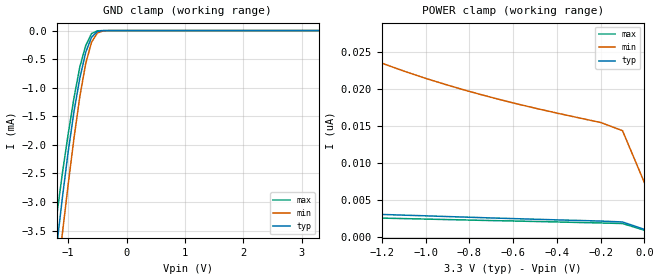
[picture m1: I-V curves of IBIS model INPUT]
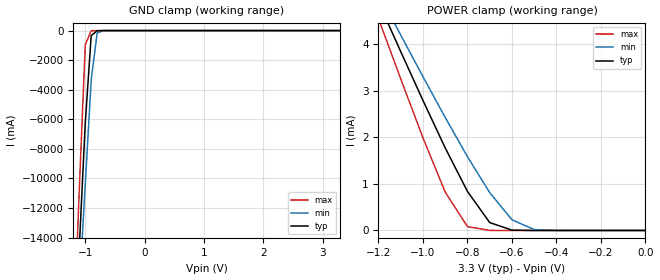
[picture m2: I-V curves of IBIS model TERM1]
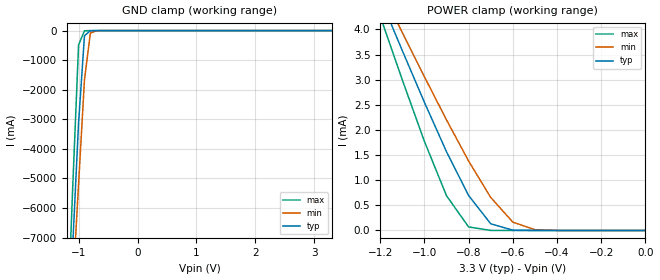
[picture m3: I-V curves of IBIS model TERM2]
|   DIODES INCORPORATED
|   IBIS Model of PI3B33X257
|   Product Family: 3B
|   BQSOP (B) Package
[IBIS Ver] 3.2
[Comment char] |_char
[File Name] pi3b33x257_b_33v.ibs
[File Rev] 1.0
[Source] File originated at Diodes Incorporated.
[Date] 10/15/15
[Disclaimer] (C) Copyright DIODES INCORPORATED
   All rights reserved
  Diodes Incorporated hereby grants the user of
  this IBIS model a non-exclusive, nontransferable license to
  use this IBIS model under the following terms.
  This IBIS model is provided on an "AS IS" basis and Diodes
  makes absolutely no warranty with respect to the information
  contained herein. DIODES DISCLAIMS AND CUSTOMER WAIVES ALL
  WARRANTIES, EXPRESSED OR IMPLIED, INCLUDING WARRANTIES OF
  MERCHANTABILITY OR FITNESS FOR A PARTICULAR PURPOSE. The
  entire risk as to quality and performance is with the customer.
  Accordingly, in no event shall the company be liable for any
  damages, whether in contract or tort, including any lost
  profits or other incidental, consequential, exemplary, or
  punitive damages arising out of the use or application of the
  IBIS model provided in this package. Further, Diodes reserves
  the right to make changes without notice to any product herein
  to improve reliability, function, or design. Diodes does not
  convey any license under patent rights or any other intellectual
  property rights, including those of third parties.
  The user is granted this license only to use the IBIS model
  and is not granted rights to sell, load, rent, lease or license
  the IBIS model in whole or in part, or in modified form to anyone
  other than user. User may modify the IBIS model to suit its specific
  application but rights to derivative works and such modifications
  shall belong to Diodes.
  Diodes is not obligated to provide maintenance or support
  for the licensed IBIS model.
  Contact Diodes at ATTN: APPLICATION ENGINEERING / IBIS MODELS
  1545 Barber Ln. Milpitas, CA 95035
[Component] PI3B33X257
[Manufacturer] Diodes Incorporated.
[Package]
| variable   typ   min   max
R_pkg   0.05665ohm   0.05080ohm   0.06250ohm
L_pkg   2.96700nH   2.48200nH   3.45200nH
C_pkg   0.32100pF   0.26800pF   0.37400pF
[Pin]   signal_name   model_name   R_pin   L_pin   C_pin
1   S0   INPUT   0.06250   3.45200nH   0.37400pF
2   IA0   TERM1   0.06144   3.36382nH   0.36436pF
3   IA1   TERM1   0.06037   3.27564nH   0.35473pF
4   YA   TERM2   0.05931   3.18745nH   0.34509pF
5   IB0   TERM1   0.05825   3.09927nH   0.33545pF
6   IB1   TERM1   0.05718   3.01109nH   0.32582pF
7   YB   TERM2   0.05612   2.92291nH   0.31618pF
8   GND   GND   0.05505   2.83473nH   0.30655pF
9   S1   INPUT   0.05399   2.74655nH   0.29691pF
10   IE0   TERM1   0.05293   2.65836nH   0.28727pF
11   IE1   TERM1   0.05186   2.57018nH   0.27764pF
12   YE   TERM2   0.05080   2.48200nH   0.26800pF
13   IF0   TERM1   0.05080   2.48200nH   0.26800pF
14   IF1   TERM1   0.05186   2.57018nH   0.27764pF
15   YF   TERM2   0.05293   2.65836nH   0.28727pF
16   GND   GND   0.05399   2.74655nH   0.29691pF
17   S2   INPUT   0.05505   2.83473nH   0.30655pF
18   II0   TERM1   0.05612   2.92291nH   0.31618pF
19   II1   TERM1   0.05718   3.01109nH   0.32582pF
20   YI   TERM2   0.05825   3.09927nH   0.33545pF
21   IJ0   TERM1   0.05931   3.18745nH   0.34509pF
22   IJ1   TERM1   0.06037   3.27564nH   0.35473pF
23   YJ   TERM2   0.06144   3.36382nH   0.36436pF
24   GND   GND   0.06250   3.45200nH   0.37400pF
25   YK   TERM2   0.06250   3.45200nH   0.37400pF
26   IK1   TERM1   0.06144   3.36382nH   0.36436pF
27   IK0   TERM1   0.06037   3.27564nH   0.35473pF
28   YL   TERM2   0.05931   3.18745nH   0.34509pF
29   IL1   TERM1   0.05825   3.09927nH   0.33545pF
30   IL0   TERM1   0.05718   3.01109nH   0.32582pF
31   _E2   INPUT   0.05612   2.92291nH   0.31618pF
32   VCC   POWER   0.05505   2.83473nH   0.30655pF
33   YG   TERM2   0.05399   2.74655nH   0.29691pF
34   IG1   TERM1   0.05293   2.65836nH   0.28727pF
35   IG0   TERM1   0.05186   2.57018nH   0.27764pF
36   YH   TERM2   0.05080   2.48200nH   0.26800pF
37   IH1   TERM1   0.05080   2.48200nH   0.26800pF
38   IH0   TERM1   0.05186   2.57018nH   0.27764pF
39   _E1   INPUT   0.05293   2.65836nH   0.28727pF
40   VCC   POWER   0.05399   2.74655nH   0.29691pF
41   YC   TERM2   0.05505   2.83473nH   0.30655pF
42   IC1   TERM1   0.05612   2.92291nH   0.31618pF
43   IC0   TERM1   0.05718   3.01109nH   0.32582pF
44   YD   TERM2   0.05825   3.09927nH   0.33545pF
45   ID1   TERM1   0.05931   3.18745nH   0.34509pF
46   ID0   TERM1   0.06037   3.27564nH   0.35473pF
47   _E0   INPUT   0.06144   3.36382nH   0.36436pF
48   VCC   POWER   0.06250   3.45200nH   0.37400pF
[Series Switch Groups]
On 1 3 5 /
Off 2 4 6 /
[Series Pin Mapping]   pin_2   model_name  function_table_group
2   4   SWITCH1   1
5   7   SWITCH1   1
43   41   SWITCH1   1
46   44   SWITCH1   1
3   4   SWITCH1   2
6   7   SWITCH1   2
42   41   SWITCH1   2
45   44   SWITCH1   2
10   12   SWITCH1   3
13   15   SWITCH1   3
35   33   SWITCH1   3
38   36   SWITCH1   3
11   12   SWITCH1   4
14   15   SWITCH1   4
34   33   SWITCH1   4
37   36   SWITCH1   4
18   20   SWITCH1   5
21   23   SWITCH1   5
27   25   SWITCH1   5
30   28   SWITCH1   5
19   20   SWITCH1   6
22   23   SWITCH1   6
26   25   SWITCH1   6
29   28   SWITCH1   6
|   Model SWITCH1
[Model] SWITCH1
Model_type Series_switch
| variable   typ   min   max
C_comp   10.500pF   10.200pF   10.800pF
[Voltage Range]   3.3000V   2.9700V   3.6300V
[GND Clamp Reference]   0.0000V   0.0000V   0.0000V
[POWER Clamp Reference]   3.3000V   2.9700V   3.6300V
[Temperature Range]   25   85   -40
[On]
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[OFF]
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| Models and submodels in the file (4): INPUT (Input), SWITCH1 (Series_switch), TERM1 (Terminator), TERM2 (Terminator)
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|   Model INPUT
[Model] INPUT
Model_type Input
Vinl = 800mV
Vinh = 2.0V
| variable   typ   min   max
C_comp   3.000pF   2.900pF   3.100pF
[Voltage Range]   3.3000V   2.9700V   3.6300V
[GND Clamp Reference]   0.0000V   0.0000V   0.0000V
[POWER Clamp Reference]   3.3000V   2.9700V   3.6300V
[Temperature Range]   25   85   -40
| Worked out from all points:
|   GND clamp passes 1 mA (typ) near -0.83 V on its own axis
[GND Clamp]
| Voltage   I(typ)   I(min)   I(max)
-3.3V     -24.17mA   -24.42mA   -24.09mA
-1.3V     -4.71mA    -5.353mA   -4.125mA
-1.2V     -3.802mA   -4.445mA   -3.269mA
-1.1V     -2.929mA   -3.554mA   -2.501mA
-1V       -2.118mA   -2.692mA   -1.809mA
-900mV    -1.411mA   -1.878mA   -1.173mA
-800mV    -829.8uA   -1.151mA   -632.5uA
-700mV    -381.7uA   -576.7uA   -263uA
-600mV    -116.2uA   -203.6uA   -52.63uA
-500mV    -16.3uA    -42uA      -3.416uA
-400mV    -1.145uA   -5.033uA   -91.97nA
3.3V      1.01nA     16.27nA    23.98pA
[POWER Clamp]   |Note: Vtable = Vcc - Voutput
| Voltage   I(typ)   I(min)   I(max)
-3.3V     6.818nA    89.17nA    3.932nA
-3V       5.933nA    71.31nA    3.74nA
-2.5V     4.813nA    49.93nA    3.389nA
-1.6V     3.476nA    28.72nA    2.808nA
-1.5V     3.356nA    27.24nA    2.739nA
-1.3V     3.13nA     24.63nA    2.602nA
-1V       2.842nA    21.42nA    2.402nA
-800mV    2.65nA     19.66nA    2.268nA
-600mV    2.465nA    18.1nA     2.143nA
-200mV    2.132nA    15.46nA    1.877nA
-100mV    2.012nA    14.35nA    1.799nA
0V        1.01nA     7.337nA    893.5pA
|   Model TERM1
[Model] TERM1
Model_type Terminator
| variable   typ   min   max
C_comp   7.000pF   6.800pF   7.200pF
[Voltage Range]   3.3000V   2.9700V   3.6300V
[GND Clamp Reference]   0.0000V   0.0000V   0.0000V
[POWER Clamp Reference]   3.3000V   2.9700V   3.6300V
[Temperature Range]   25   85   -40
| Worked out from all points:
|   GND clamp passes 1 mA (typ) near -0.71 V on its own axis
|   POWER clamp passes 1 mA (typ) near -0.82 V on its own axis
[GND Clamp]
| Voltage   I(typ)   I(min)   I(max)
-3.3V     -198.2A    -172.9A    -239.3A
-1.2V     -22.95A    -24.52A    -21.07A
-1.1V     -14.6A     -17.46A    -10.67A
-1V       -6.255A    -10.4A     -968.6mA
-900mV    -345.5mA   -3.339A    -11.3mA
-800mV    -10.61mA   -172.3mA   -151.5uA
-700mV    -350.4uA   -9.392mA   -1.276uA
3.3V      786.5pA    112.3nA    110.4pA
[POWER Clamp]   |Note: Vtable = Vcc - Voutput
| Voltage   I(typ)   I(min)   I(max)
-3.3V     26.63mA    24.59mA    29.73mA
-1.2V     4.898mA    5.094mA    4.542mA
-1.1V     3.836mA    4.191mA    3.25mA
-1V       2.787mA    3.298mA    1.985mA
-900mV    1.77mA     2.423mA    821.9uA
-800mV    836.8uA    1.582mA    82.7uA
-700mV    169.7uA    811.8uA    826.1nA
-600mV    6.664uA    229.3uA    8.305nA
-500mV    147.7nA    20.06uA    2.399nA
-400mV    5.577nA    918.8nA    2.265nA
0V        786.5pA    4.94nA     722pA
|   Model TERM2
[Model] TERM2
Model_type Terminator
| variable   typ   min   max
C_comp   3.500pF   3.4000pF   3.600pF
[Voltage Range]   3.3000V   2.9700V   3.6300V
[GND Clamp Reference]   0.0000V   0.0000V   0.0000V
[POWER Clamp Reference]   3.3000V   2.9700V   3.6300V
[Temperature Range]   25   85   -40
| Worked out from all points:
|   GND clamp passes 1 mA (typ) near -0.71 V on its own axis
|   POWER clamp passes 1 mA (typ) near -0.83 V on its own axis
[GND Clamp]
| Voltage   I(typ)   I(min)   I(max)
-3.3V     -99.12A    -86.44A    -119.7A
-1.2V     -11.47A    -12.26A    -10.53A
-1.1V     -7.301A    -8.73A     -5.338A
-1V       -3.129A    -5.2A      -486.2mA
-900mV    -174.2mA   -1.671A    -6.956mA
-800mV    -6.311mA   -87.22mA   -146.7uA
-700mV    -315.8uA   -5.394mA   -1.275uA
3.3V      730.4pA    102.9nA    65.03pA
[POWER Clamp]   |Note: Vtable = Vcc - Voutput
| Voltage   I(typ)   I(min)   I(max)
-3.3V     26.24mA    24.2mA     29.33mA
-1.2V     4.628mA    4.834mA    4.266mA
-1.1V     3.58mA     3.941mA    2.998mA
-1V       2.552mA    3.06mA     1.774mA
-900mV    1.567mA    2.201mA    692.7uA
-800mV    695.9uA    1.383mA    70.32uA
-700mV    133.2uA    657.6uA    811.8nA
-600mV    6.007uA    166.8uA    8.287nA
-500mV    143.5nA    15.36uA    2.397nA
0V        730.8pA    4.881nA    663pA
